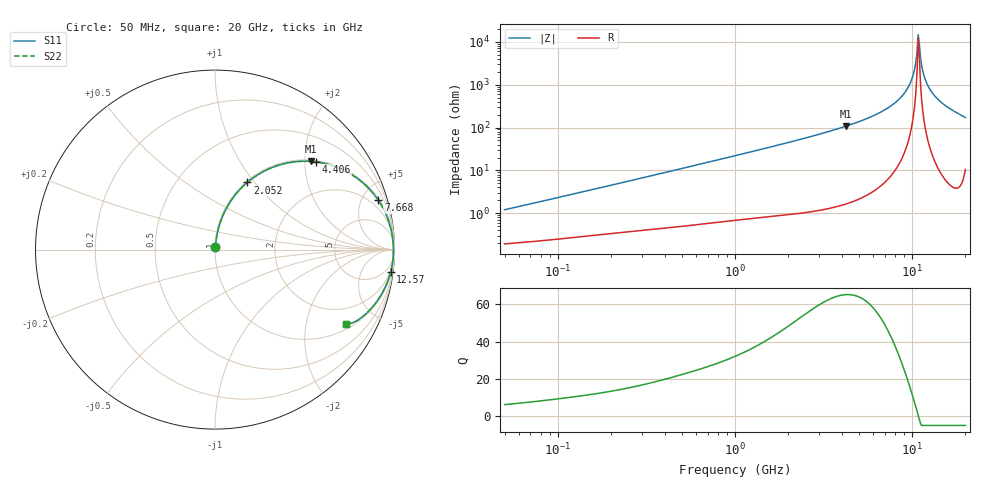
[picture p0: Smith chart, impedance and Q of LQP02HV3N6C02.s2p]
!Murata Part Number: LQP02HV3N6C02
!These Parameters are Measured in Series Mode Connection
!  o--[Z]--o
!Port1  Port2
!  o-------o
!Freq. Start=50[MHz] Stop=20[GHz], 401[Steps]
# Hz S RI R 50
!Freq.(Hz) S11(Real) S11(Imag) S21(Real) S21(Imag) S12(Real) S12(Imag) S22(Real) S22(Imag)
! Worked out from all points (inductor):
!   401 points, 50 MHz to 20 GHz, reference 50 ohm
!   read as one part in series: L = 3.76 nH near 51.52 MHz
!   highest Q = 65.2 at 4.212 GHz (marker M1), where L = 4.04 nH
!   self-resonance near 10.82 GHz
!   S11 on the Smith chart (normalised r, x): 50 MHz: 1.00, +0.02; 2.052 GHz: 1.02, +0.92; 4.406 GHz: 1.03, +2.27; 7.668 GHz: 1.16, +6.57; 12.57 GHz: 2, -16; 20 GHz: 1.21, -3.41
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5e7  0.00207 0.0119  0.9979 -0.0119  0.9979 -0.0119  0.00207 0.0119
1.364002e8  0.00382 0.031  0.9962 -0.031  0.9962 -0.031  0.00382 0.031
3.721004e8  0.011 0.0814  0.989 -0.0814  0.989 -0.0814  0.011 0.0814
1e9  0.052 0.207  0.948 -0.207  0.948 -0.207  0.052 0.207
2.05233e9  0.1797 0.3739  0.8203 -0.3739  0.8203 -0.3739  0.1797 0.3739
2.728004e9  0.2865 0.4435  0.7135 -0.4435  0.7135 -0.4435  0.2865 0.4435
4.212059e9  0.5324 0.4913  0.4676 -0.4913  0.4676 -0.4913  0.5324 0.4913
4.405649e9  0.5625 0.4885  0.4375 -0.4885  0.4375 -0.4885  0.5625 0.4885
5.944466e9  0.7655 0.4152  0.2345 -0.4152  0.2345 -0.4152  0.7655 0.4152
7.442007e9  0.8956 0.2948  0.1044 -0.2948  0.1044 -0.2948  0.8956 0.2948
7.668323e9  0.9098 0.2748  0.0902 -0.2748  0.0902 -0.2748  0.9098 0.2748
8.774992e9  0.9612 0.1761  0.0388 -0.1761  0.0388 -0.1761  0.9612 0.1761
9.600142e9  0.9829 0.1039  0.0171 -0.1039  0.0171 -0.1039  0.9829 0.1039
1.019291e10  0.9911 0.054  0.00889 -0.054  0.00889 -0.054  0.9911 0.054
1.066139e10  0.9939 0.0161  0.00608 -0.0161  0.00608 -0.0161  0.9939 0.0161
1.082228e10  0.9942 0.00343  0.00579 -0.00343  0.00579 -0.00343  0.9942 0.00343
1.115139e10  0.9938 -0.022  0.00619 0.022  0.00619 0.022  0.9938 -0.022
1.149051e10  0.9921 -0.0473  0.00789 0.0473  0.00789 0.0473  0.9921 -0.0473
1.166392e10  0.9908 -0.0599  0.00923 0.0599  0.00923 0.0599  0.9908 -0.0599
1.257102e10  0.9792 -0.1223  0.0208 0.1223  0.0208 0.1223  0.9792 -0.1223
1.504638e10  0.9202 -0.2613  0.0798 0.2613  0.0798 0.2613  0.9202 -0.2613
2e10  0.732 -0.4131  0.268 0.4131  0.268 0.4131  0.732 -0.4131
